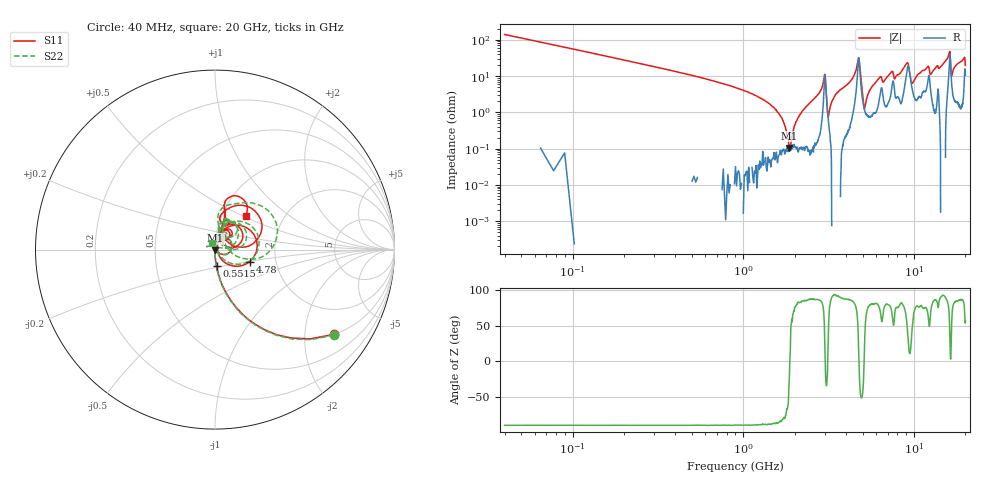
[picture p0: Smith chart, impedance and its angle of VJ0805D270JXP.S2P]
! VJ0805D270JXP
! DATE 10/29/2021  12:24
! CAPACITORS MOUNTED IN SERIES ON 25 MIL THICK MICROSTRIP SUBSTRATE
# GHz  S  MA  R  50.00
!  FREQ  S11M  S11A  S21M  S21A  S12M  S12A  S22M  S22A
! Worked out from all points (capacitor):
!   1601 points, 40 MHz to 20 GHz, reference 50 ohm
!   read as one part in series: C = 28.3 pF near 139.8 MHz
!   lowest |Z| = 105 mohm at 1.861 GHz (marker M1)
!   series resonance near 1.874 GHz, so ESL is about 250 pH
!   S11 on the Smith chart (normalised r, x): 40 MHz: 1.00, -2.79; 551.5 MHz: 1.00, -0.19; 4.78 GHz: 1.46, -0.20; 20 GHz: 1.29, +0.52
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0.04  0.8123 -35.6  0.5795 54.5  0.5786 54.3  0.8169 -35.6
0.21465  0.2498 -75.4  0.9683 14.5  0.9682 14.4  0.2527 -75.9
0.551475  0.09329 -84.6  0.9949 5.3  0.9959 5.3  0.09521 -85.2
1.524525  0.01541 -87.8  0.9987 0.6  0.9996 0.5  0.0161 -87.1
1.86135  0.003786 -74.4  0.9988 -0.1  0.9992 -0.2  0.003698 -75.6
2.01105  0.00125 65.4  0.9985 -0.4  0.9988 -0.5  0.0014 31.7
2.946675  0.06263 67.7  0.9781 -4.0  0.9794 -4.1  0.06327 69.2
3.1837  0.007281 24.7  0.9954 -0.8  0.997 -0.9  0.004442 75.9
3.370825  0.01485 81.7  1 -1.7  1.001 -1.9  0.01982 103.3
4.7805  0.2049 -19.1  0.7955 3.1  0.7968 3.0  0.2183 -11.5
5.1797  0.01368 10.2  0.99 -1.1  0.9905 -1.2  0.007903 37.6
5.75355  0.04259 64.5  0.9891 -3.5  0.9905 -3.7  0.05395 85.3
6.70165  0.06674 65.9  0.9814 -4.5  0.9811 -4.6  0.06258 74.7
9.109325  0.1829 37.9  0.8611 -9.6  0.8622 -9.8  0.2025 39.7
9.69565  0.06013 22.7  0.9484 -2.8  0.9498 -2.9  0.04744 27.9
10.02  0.06475 52.8  0.9716 -4.7  0.9725 -4.9  0.06145 71.1
11.37978  0.08716 55.8  0.9553 -8.2  0.9563 -8.4  0.1669 70.9
13.35083  0.1484 72.9  0.9776 -10.4  0.9786 -10.7  0.1439 80.2
16.13275  0.3092 44.6  0.7625 -19.2  0.7635 -19.6  0.372 28.4
16.68165  0.08319 50.2  0.9476 -6.8  0.9486 -7.1  0.0732 48.8
19.57585  0.2838 77.3  0.9113 -19.9  0.9123 -20.0  0.1794 51.5
20  0.2528 47.6  0.8545 -10.5  0.8554 -10.9  0.03964 115.0
